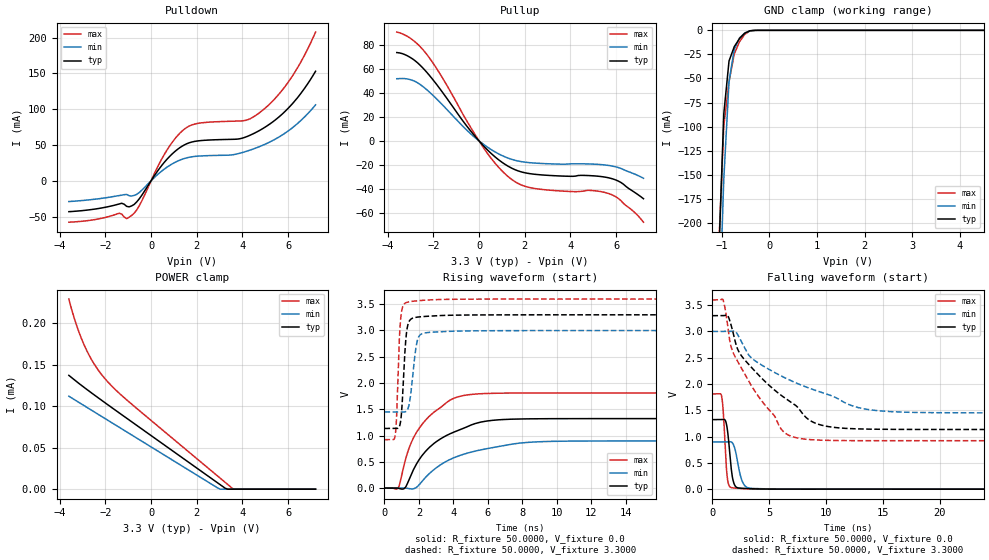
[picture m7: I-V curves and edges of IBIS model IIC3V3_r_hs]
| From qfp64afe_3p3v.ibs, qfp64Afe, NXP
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[Model] IIC3V3_r_hs
|   Model IIC3V3_r_hs
| This model was characterised for following simulation conditions:
| External (pad) voltage:
|   - Typ: 3.3V,   - Min: 3.0V,   - Max: 3.6V
| Library cells for typ/min/max conditions are connected as defined below:
|  IO - External Pad
|  A - Core Input
|  EN - Output Buffer Enable
|  BOOST - vdde
|  EGP - vdd
|  EHS - vdd
|  ENZI - vdd
|  EPD - vdd
|  EPUN - gnd
|  ZI - NC
|  ZIF - NC
|  gnd - gnd
|  gnde - gnde
|  vdd - vdd
|  vdde - vdde
| All other pins connected to ground
Model_type I/O
Polarity   Non-Inverting
Enable   Active-Low
Vinl =   0.9900V
Vinh =   2.3100V
Vmeas =  1.6500V
Cref =   0.0F
Rref =   1.0000k
Vref =   0.0V
C_comp   3.5907pF   3.4406pF   3.7387pF
|C_comp_pullup   0.9138pF   0.9000pF   0.9174pF
|C_comp_pulldown   2.3267pF   2.4802pF   2.1806pF
[Model Spec]
| variable   typ   min   max
Vinh   0.9900V   0.9000V   1.0800V
Vinl   2.3100V   2.1000V   2.5200V
Vmeas   1.6500V   1.5000V   1.8000V
[Temperature Range]   25.0000   0.1250k   -40.0000
[Voltage Range]   3.3000V   3.0000V   3.6000V
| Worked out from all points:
|   slope of the pulldown table from 0 to 0.495 V, typ, clamps not added: 22 ohm
|   slope of the pullup table from 0 to 0.495 V, typ, clamps not added: 50.2 ohm
|   GND clamp passes 1 mA (typ) near -0.43 V on its own axis
|   rising waveform, R_fixture 50.0000, V_fixture 0.0: 20-80 % time 2.42ns typ, 3.15ns min, 1.81ns max; typ from 0 V to 1.32 V
|   rising waveform, R_fixture 50.0000, V_fixture 3.3000: 20-80 % time 230ps typ, 322ps min, 186ps max; typ from 1.14 V to 3.3 V
|   falling waveform, R_fixture 50.0000, V_fixture 0.0: 20-80 % time 371ps typ, 533ps min, 281ps max; typ from 1.32 V to 0 V
|   falling waveform, R_fixture 50.0000, V_fixture 3.3000: 20-80 % time 5.5ns typ, 7.83ns min, 3.83ns max; typ from 3.3 V to 1.14 V
[Pulldown]
|Voltage   I(typ)   I(min)   I(max)
-3.6V     -43.22mA   -29.09mA   -57.9mA
-1.29V    -31.46mA   -20.15mA   -46.47mA
-1.07V    -35.79mA   -19.19mA   -52.9mA
-850mV    -35.14mA   -21.36mA   -48.43mA
-520mV    -25.35mA   -16.52mA   -35.11mA
580mV     25.81mA    16.3mA     36.8mA
1.24V     45.79mA    28.53mA    65.82mA
1.9V      54.89mA    33.9mA     79.08mA
4.1V      60.55mA    40.38mA    84.05mA
4.76V     70.44mA    47.87mA    95.32mA
6.08V     103.9mA    71.39mA    141.2mA
7.2V      152.9mA    106mA      207.6mA
[Pullup]
|Voltage   I(typ)   I(min)   I(max)
-3.6V     73.65mA    51.83mA    90.73mA
-2.92V    68.52mA    50.55mA    84.41mA
-2.26V    56.61mA    42.22mA    71.46mA
-1.6V     40.53mA    30.04mA    52.53mA
160mV     -3.403mA   -2.371mA   -4.704mA
820mV     -15.2mA    -10.46mA   -21.22mA
1.37V     -22.16mA   -15.02mA   -31.28mA
1.81V     -25.65mA   -17.18mA   -36.45mA
2.47V     -27.92mA   -18.56mA   -39.79mA
5.66V     -30.76mA   -20.47mA   -43.83mA
6.1V      -33.55mA   -22.29mA   -48.04mA
7.2V      -48.27mA   -31.2mA    -67.82mA
[GND_clamp]
|Voltage   I(typ)   I(min)   I(max)
-3.6V     -5.602A    -5.487A    -5.717A
-1.07V    -242mA     -316.8mA   -230.5mA
-960mV    -86.76mA   -154.7mA   -99.49mA
-850mV    -31.82mA   -53.09mA   -53.51mA
-740mV    -16.97mA   -19.87mA   -24.44mA
-630mV    -8.597mA   -7.926mA   -11.89mA
-520mV    -3.004mA   -2.733mA   -4.196mA
-410mV    -439.7uA   -501.8uA   -589.4uA
7.2V      0A         0A         0A
[POWER_clamp]
|Voltage   I(typ)   I(min)   I(max)
-3.6V     137uA      111.9uA    228.9uA
-3.47V    134.1uA    109.7uA    215.6uA
-3.25V    129.3uA    106uA      196.2uA
-2.92V    122.3uA    100.4uA    172.9uA
-2.48V    113.3uA    92.88uA    150.2uA
-2.04V    104.5uA    85.42uA    133.7uA
-1.16V    87.2uA     70.51uA    109.7uA
2.91V     7.626uA    1.527uA    15.86uA
3.02V     5.475uA    0A         13.33uA
3.24V     1.173uA    0A         8.273uA
3.57V     0A         0A         687.1nA
7.2V      0A         0A         0A
[Ramp]
| variable   typ   min   max
dV/dt_r  0.7935/2.4156n   0.5386/3.1486n   1.0867/1.8102n
dV/dt_f  1.2983/5.5029n   0.9293/7.8321n   1.6062/3.8295n
R_load = 50.0000
[Rising Waveform]
R_fixture= 50.0000
V_fixture= 0.0
V_fixture_min= 0.0
V_fixture_max= 0.0
|time   V(typ)   V(min)   V(max)
0s        2.145nV    50.58nV    26.14nV
791.5ps   -3mV       53.96uV    -88.64uV
1.203ns   7.776mV    -1.263mV   521.6mV
1.483ns   203.5mV    -14.57mV   808.1mV
1.808ns   428.2mV    1.866mV    1.031V
2.635ns   782mV      284.2mV    1.377V
3.689ns   1.015V     525.5mV    1.649V
5.623ns   1.258V     729.2mV    1.796V
7.659ns   1.314V     848.4mV    1.809V
1us       1.322V     897.6mV    1.811V
[Rising Waveform]
R_fixture= 50.0000
V_fixture= 3.3000
V_fixture_min= 3.0000
V_fixture_max= 3.6000
|time   V(typ)   V(min)   V(max)
0s        1.135V     1.45V      921.3mV
628.5ps   1.134V     1.45V      1.014V
702ps     1.133V     1.45V      1.334V
905.8ps   1.211V     1.449V     3.078V
1.104ns   2.076V     1.447V     3.485V
1.224ns   2.764V     1.453V     3.525V
1.357ns   3.104V     1.506V     3.541V
2.027ns   3.259V     2.901V     3.569V
4.449ns   3.294V     2.99V      3.596V
1us       3.299V     2.999V     3.598V
[Falling Waveform]
R_fixture= 50.0000
V_fixture= 0.0
V_fixture_min= 0.0
V_fixture_max= 0.0
|time   V(typ)   V(min)   V(max)
0s        1.322V     897.6mV    1.811V
824ps     1.322V     897.6mV    1.754V
976.2ps   1.325V     897.6mV    1.416V
1.256ns   1.216V     897.5mV    337.7mV
1.481ns   803mV      899.7mV    61.82mV
1.724ns   277.8mV    888.8mV    26.97mV
2.018ns   56.81mV    737.3mV    19.16mV
2.771ns   14.25mV    89.62mV    10.36mV
4.253ns   3.26mV     7.368mV    1.632mV
1us       13.83nV    70.96nV    33.33nV
[Falling Waveform]
R_fixture= 50.0000
V_fixture= 3.3000
V_fixture_min= 3.0000
V_fixture_max= 3.6000
|time   V(typ)   V(min)   V(max)
0s        3.299V     2.999V     3.598V
923.9ps   3.298V     2.999V     3.606V
1.371ns   3.293V     2.998V     3.066V
1.863ns   2.94V      3.008V     2.577V
2.639ns   2.511V     2.769V     2.267V
6.138ns   1.77V      2.143V     1.119V
10.86ns   1.171V     1.74V      925mV
14.56ns   1.139V     1.492V     921.7mV
23.45ns   1.135V     1.451V     921.4mV
1us       1.135V     1.45V      921.3mV
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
